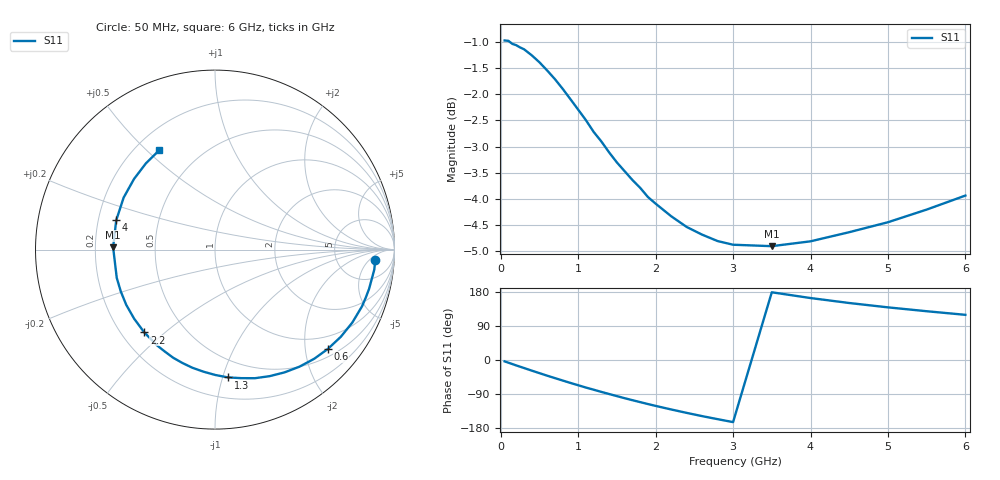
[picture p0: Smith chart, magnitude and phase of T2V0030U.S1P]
! SIEMENS Discrete & RF Semiconductors
! BAS70-04W
! Si Schottky Diode in SOT323
! IF = 0.03 mA
! S-Parameters:  November  1997
# GHz  S  MA  R  50
!  f  S11
! GHz  MAG  ANG
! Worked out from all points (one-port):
!   34 points, 50 MHz to 6 GHz, reference 50 ohm
!   lowest |S11| = -4.9 dB at 3.5 GHz (marker M1), VSWR 3.63, Z = 13.8 + j0.524 ohm
!   |S11| at or under -10 dB: nowhere
!   S11 on the Smith chart (normalised r, x): 50 MHz: 14, -8; 600 MHz: 0.67, -2.49; 1.3 GHz: 0.36, -1.04; 2.2 GHz: 0.29, -0.43; 4 GHz: 0.28, +0.13; 6 GHz: 0.29, +0.55
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0.05  0.8952 -3.6
0.1  0.8944 -7.2
0.2  0.8859 -14.3
0.3  0.878 -21.1
0.4  0.8663 -28.0
0.5  0.8529 -34.7
0.6  0.8376 -41.4
0.7  0.8217 -47.8
0.8  0.8043 -54.2
0.9  0.7861 -60.5
1  0.7681 -66.6
1.1  0.7504 -72.7
1.3  0.7158 -84.2
1.4  0.6987 -89.8
1.6  0.6703 -100.8
1.8  0.6461 -111.1
1.9  0.6331 -116.2
2  0.6239 -121.1
2.2  0.6068 -130.5
2.4  0.5925 -139.5
2.6  0.5825 -148.1
3  0.5696 -163.9
3.5  0.5678 178.7
4  0.574 163.5
4.5  0.5857 150.4
5  0.5987 138.9
5.5  0.6157 128.7
6  0.6351 119.2
